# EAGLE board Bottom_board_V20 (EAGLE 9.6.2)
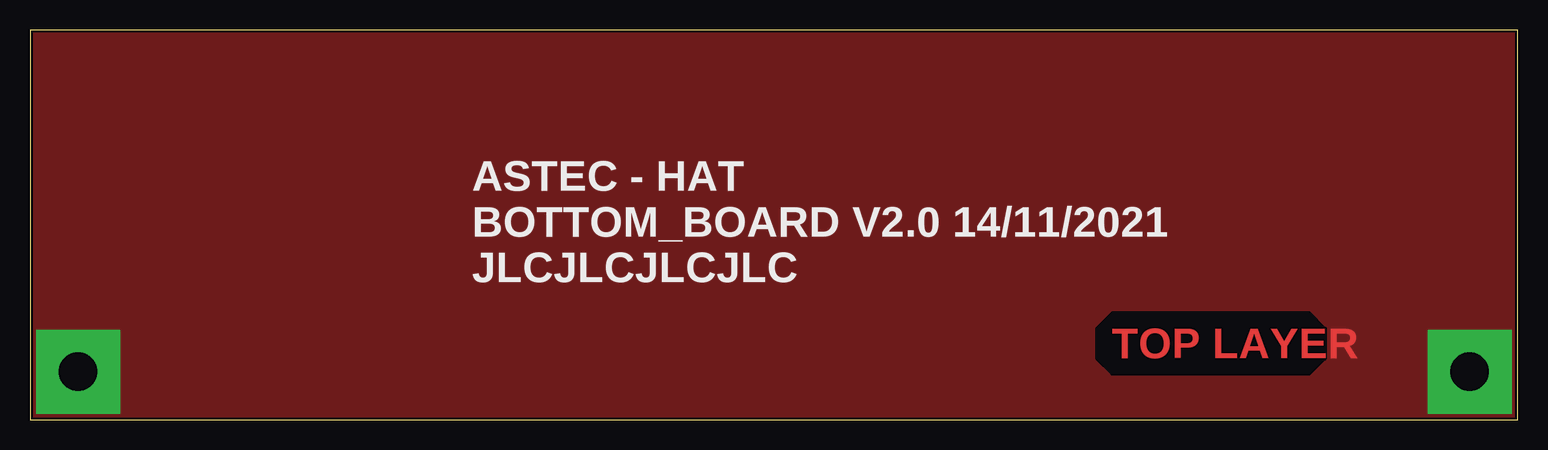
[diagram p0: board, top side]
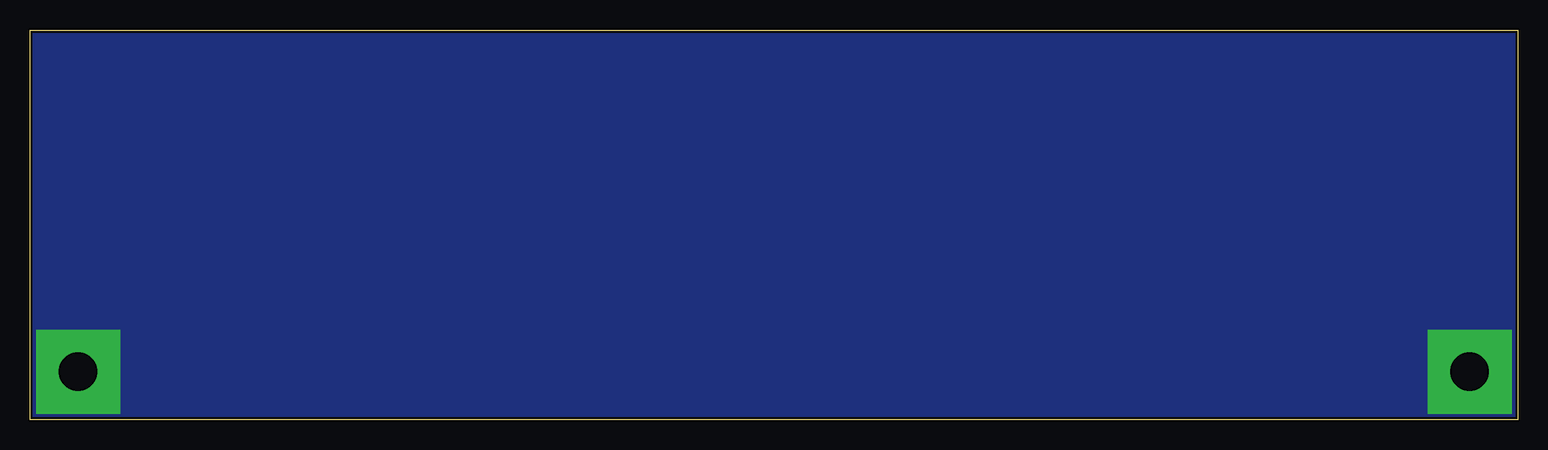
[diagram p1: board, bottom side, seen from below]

Size 124 x 32.5 mm. Coordinates in mm from the lower left corner, seen from the top.
Outline: 0,0 124,0 124,32.5 0,32.5 0,0
Copper layers (1*16): Top 0.035mm / dielectric 1.5mm / Bottom 0.035mm
Design rules "JLCPCB_2alyer": minimum track width 5mil, minimum drill 0.2mm, track to track 5mil, track to pad 0.2mm, pad to pad 0.2mm, via to via 0.2mm, smd to smd 5mil, copper to edge 0.2mm, drill to drill 0.5mm, minimum pad ring 0.13mm, minimum via ring 0.13mm, stop-mask expansion 0.05mm, vias tented up to drill 0mil, thermal gap 10mil
tRestrict: 8 lines

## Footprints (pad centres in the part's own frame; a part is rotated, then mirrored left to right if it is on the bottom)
M-PAD_M3(POLYGON) = drill 3.2 pad 7 square: P$1 0,0

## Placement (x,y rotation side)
P1  M-PAD_M3(POLYGON)  [M-PAD_M3(POLYGON)]  4,4 0 top
P2  M-PAD_M3(POLYGON)  [M-PAD_M3(POLYGON)]  120,4 0 top

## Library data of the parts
P1 P2 = Antec-Hood

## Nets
GND: P1.P$1 P2.P$1

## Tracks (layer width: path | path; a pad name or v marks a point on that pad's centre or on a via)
GND
  pour Top (no thermals): -1.27,34.29 -1.27,-1.27 0,-2.54 125.73,-2.54 127,-1.27 127,35.56 1.27,35.56 0,35.56
  pour Bottom (no thermals): -1.27,36.83 -1.27,-3.81 0,-5.08 125.73,-5.08 127,-3.81 127,36.83 125.73,38.1 0,38.1

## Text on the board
Top: TOP LAYER
tPlace: ASTEC - HAT / BOTTOM_BOARD V2.0 14/11/2021 / JLCJLCJLCJLC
